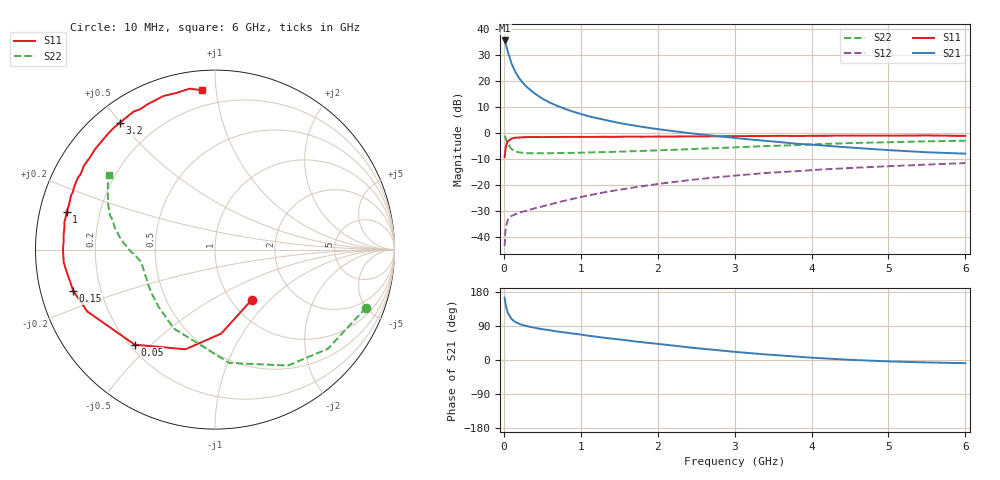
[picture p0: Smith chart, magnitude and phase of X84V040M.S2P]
! SIEMENS Small Signal Semiconductors
! BFP136W
! Si NPN RF Bipolar Junction Transistor in SOT343
! VCE = 4 V  IC = 40 mA
! Common Emitter S-Parameters:  September  1994
# GHz  S  MA  R  50
!  f  S11  S21  S12  S22
! GHz  MAG  ANG  MAG  ANG  MAG  ANG  MAG  ANG
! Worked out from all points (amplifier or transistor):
!   40 points, 10 MHz to 6 GHz, reference 50 ohm
!   highest |S21| = 35.6 dB at 10 MHz (marker M1)
!   |S21| within 3 dB of that: start of sweep to 39.78 MHz
!   unconditionally stable (mu >= 1): 738.2 MHz to 2.835 GHz
!   at 200 MHz: K = 0.48, MSG = 25.8 dB, |S12| = -30.4 dB
!   at 1.5 GHz: K = 1.11, MAG = 10.8 dB, |S12| = -21.7 dB
!   at 6 GHz: K = 0.96, MSG = 1.8 dB, |S12| = -11.5 dB
!   S11 on the Smith chart (normalised r, x): 10 MHz: 1.24, -0.79; 50 MHz: 0.22, -0.45; 150 MHz: 0.10, -0.14; 1 GHz: 0.08, +0.12; 3.2 GHz: 0.08, +0.50; 6 GHz: 0.11, +0.92
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0.01  0.3468 -53.8  60.54 164.7  0.0068 74.0  0.9018 -21.0
0.02  0.4694 -85.8  54.71 151.1  0.0126 63.1  0.8372 -41.3
0.03  0.5794 -106.5  48.92 140.2  0.0165 54.0  0.7634 -57.8
0.05  0.6935 -130.2  37.33 125.2  0.0217 41.9  0.6365 -82.8
0.1  0.7904 -154.1  21.81 108.0  0.0259 32.2  0.4956 -117.7
0.15  0.8227 -163.8  15.05 100.1  0.0279 31.3  0.447 -134.9
0.2  0.829 -168.7  11.38 95.4  0.0301 31.1  0.4297 -144.9
0.25  0.8392 -172.8  9.198 91.9  0.0314 32.6  0.4215 -151.2
0.3  0.8457 -175.2  7.705 89.4  0.0326 34.9  0.4155 -155.6
0.4  0.8471 180.0  5.811 84.9  0.0363 38.5  0.4136 -161.3
0.5  0.8447 176.8  4.636 81.3  0.0394 41.4  0.4133 -164.9
0.6  0.8474 174.5  3.866 78.4  0.043 44.4  0.4145 -167.1
0.7  0.848 171.6  3.333 75.0  0.047 47.0  0.4165 -168.6
0.8  0.8529 169.9  2.915 72.5  0.0512 49.0  0.4185 -170.0
1  0.8529 165.9  2.353 67.2  0.0597 51.9  0.4243 -172.0
1.1  0.8509 163.1  2.129 63.9  0.064 52.7  0.4279 -172.7
1.5  0.8582 156.4  1.577 54.2  0.0823 54.8  0.4432 -175.3
2.2  0.8654 143.9  1.1 38.1  0.1155 53.2  0.4809 179.6
3.2  0.884 126.9  0.761 18.1  0.1628 46.0  0.5507 170.3
4.5  0.9029 108.5  0.533 0.5  0.2154 34.6  0.6483 156.8
5.5  0.9079 99.0  0.432 -6.4  0.2506 26.8  0.7003 148.5
6  0.8908 94.7  0.406 -8.5  0.2675 22.3  0.7194 144.9
